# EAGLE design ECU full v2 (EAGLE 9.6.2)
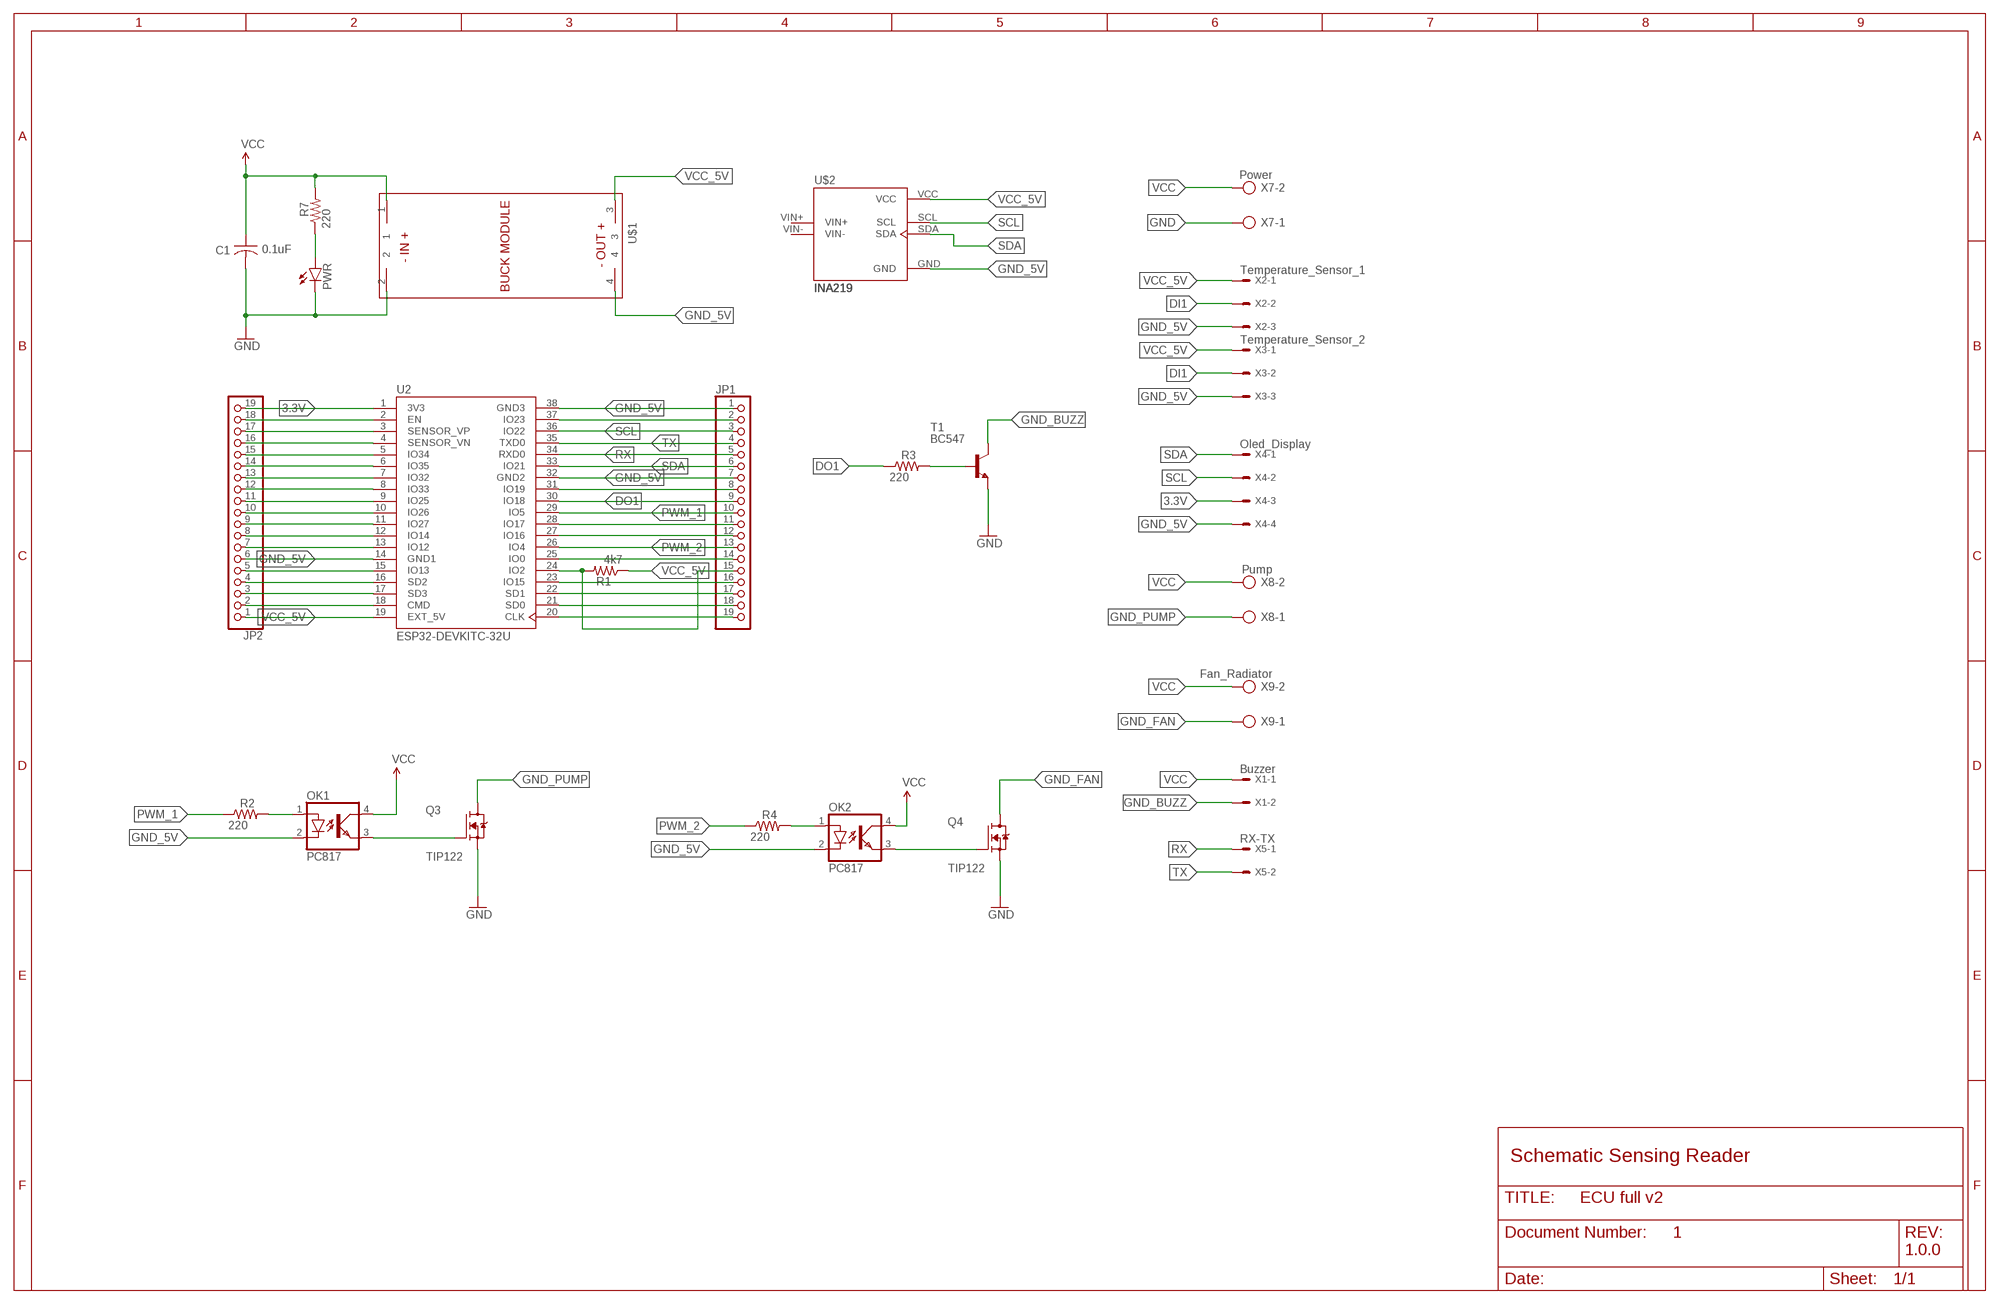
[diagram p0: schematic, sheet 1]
FRAME1 (FRAME_B_L): DESIGNER: PRATIK MAKWANA; DOC: 1; REV: 1.0.0

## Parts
C1  0.1uF  C-US050-030X075  [C050-030X075]
JP1  PINHD-1X19  [1X19]
JP2  PINHD-1X19  [1X19]
OK1  PC817  [DIL04]
OK2  PC817  [DIL04]
PWR  LED5MM  [LED5MM]
Q3  TIP122  IRF3205  [TO254P1041X444X2933-3]
Q4  TIP122  IRF3205  [TO254P1041X444X2933-3]
R1  4k7  R-US_0207/10  [0207/10]
R2  220  R-US_0207/10  [0207/10]
R3  220  R-US_0207/10  [0207/10]
R4  220  R-US_0207/10  [0207/10]
R7  220  R-US_0207/10  [0207/10]
T1  BC547  [TO92]
U2  ESP32-DEVKITC-32U  [MODULE_ESP32-DEVKITC-32U]
U$1  BUCK_MODULEWITH_SMDPADS&THROUGHHOLES  [BUCK_MODULE]
U$2  INA219  [INA219]
X1  Buzzer  22-23-2021  [22-23-2021]
X2  Temperature_Sensor_1  22-23-2031  [22-23-2031]
X3  Temperature_Sensor_2  22-23-2031  [22-23-2031]
X4  Oled_Display  22-23-2041  [22-23-2041]
X5  RX-TX  22-23-2021  [22-23-2021]
X7  Power  AK500/2  [AK500/2]
X8  Pump  AK500/2  [AK500/2]
X9  Fan_Radiator  AK500/2  [AK500/2]

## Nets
3.3V: JP2.19 U2.1(3V3) X4.3
DI1: JP1.15 R1.2 U2.24(IO2) X2.2 X3.2
DO1: JP1.9 R3.1 U2.30(IO18)
GND: C1.2 PWR.K(C) Q3.3(S) Q4.3(S) T1.1(E) U$1.2 X7.1
GND_5V: JP1.1 JP1.7 JP2.6 OK1.2(C) OK2.2(C) U2.14(GND1) U2.32(GND2) U2.38(GND3) U$1.4 U$2.GND X2.3 X3.3 X4.4
GND_BUZZ: T1.3(C) X1.2
GND_FAN: Q4.2(D) X9.1
GND_PUMP: Q3.2(D) X8.1
N$1: OK1.1(A) R2.2
N$2: JP2.18 U2.2(EN)
N$3: JP2.17 U2.3(SENSOR_VP)
N$4: JP2.16 U2.4(SENSOR_VN)
N$5: JP2.15 U2.5(IO34)
N$6: JP2.14 U2.6(IO35)
N$7: JP2.13 U2.7(IO32)
N$8: JP2.12 U2.8(IO33)
N$9: JP2.11 U2.9(IO25)
N$10: JP2.10 U2.10(IO26)
N$11: JP2.9 U2.11(IO27)
N$12: JP2.8 U2.12(IO14)
N$13: JP2.7 U2.13(IO12)
N$14: JP2.5 U2.15(IO13)
N$15: OK1.3(EMIT) Q3.1(G)
N$16: OK2.1(A) R4.2
N$17: OK2.3(EMIT) Q4.1(G)
N$18: JP1.19 U2.20(CLK)
N$19: JP1.18 U2.21(SD0)
N$20: JP1.17 U2.22(SD1)
N$21: JP1.14 U2.25(IO0)
N$22: JP1.16 U2.23(IO15)
N$23: JP1.12 U2.27(IO16)
N$24: JP1.11 U2.28(IO17)
N$25: JP2.2 U2.18(CMD)
N$26: JP1.2 U2.37(IO23)
N$27: JP2.3 U2.17(SD3)
N$28: JP2.4 U2.16(SD2)
N$29: JP1.8 U2.31(IO19)
N$30: PWR.A R7.1
N$33: R3.2 T1.2(B)
PWM_1: JP1.10 R2.1 U2.29(IO5)
PWM_2: JP1.13 R4.1 U2.26(IO4)
RX: JP1.5 U2.34(RXD0) X5.1
SCL: JP1.3 U2.36(IO22) U$2.SCL X4.2
SDA: JP1.6 U2.33(IO21) U$2.SDA X4.1
TX: JP1.4 U2.35(TXD0) X5.2
VCC: C1.1 OK1.4(COL) OK2.4(COL) R7.2 U$1.1 X1.1 X7.2 X8.2 X9.2
VCC_5V: JP2.1 R1.1 U2.19(EXT_5V) U$1.3 U$2.VCC X2.1 X3.1
Unconnected: U$2.VIN+ U$2.VIN-

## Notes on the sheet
- Schematic Sensing Reader

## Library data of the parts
C1 = adafruit:C-US: CAPACITOR, American symbol
JP1 JP2 = pinhead:PINHD-1X19: PIN HEADER
OK1 OK2 = optocoupler:PC817: SHARP OPTO COUPLER; MPN: PC817X4J000F; OC_FARNELL: 9707727; OC_NEWARK: 97K7059
PWR = led:LED: LED
Q3 Q4 = IRF3205:IRF3205: N-Channel 55V 75A (Tc) 170W (Tc) Through Hole TO-220AB Check availability; AVAILABILITY: In Stock; CHECK_PRICES: https://www.snapeda.com/parts/IRF3205/Infineon/view-part/?ref=eda; DESCRIPTION: N-Channel 55V 110A (Tc) 200W (Tc) Through Hole TO-220AB; MF: Infineon Technologies; MP: IRF3205; PACKAGE: TO-220 Infineon; PRICE: None; SNAPEDA_LINK: https://www.snapeda.com/parts/IRF3205/Infineon/view-part/?ref=snap
R1-R4 R7 = adafruit:R-US_: RESISTOR, American symbol
T1 = transistor:BC547: NPN TRANSISTOR
U2 = ESP32-DEVKITC-32U:ESP32-DEVKITC-32U: Check availability; AVAILABILITY: In Stock; CHECK_PRICES: https://www.snapeda.com/parts/ESP32-DEVKITC-32U/Espressif+Systems/view-part/?ref=eda; DESCRIPTION: ESP32-WROOM-32UE series Transceiver; 802.11 b/g/n (Wi-Fi, WiFi, WLAN), Bluetooth® Smart Ready 4.x Dual Mode Evaluation Board; MF: Espressif Systems; MP: ESP32-DEVKITC-32U; PACKAGE: CUSTOM-38 ESPRESSIF; PRICE: None; SNAPEDA_LINK: https://www.snapeda.com/parts/ESP32-DEVKITC-32U/Espressif+Systems/view-part/?ref=snap
U$1 = BUCK_MODULE:BUCK_MODULE
U$2 = INA219:INA219
X1 X5 = con-molex:22-23-2021: .100" (2.54mm) Center Header - 2 Pin; MF: MOLEX; MPN: 22-23-2021; OC_FARNELL: 1462926; OC_NEWARK: 25C3832
X2 X3 = con-molex:22-23-2031: .100" (2.54mm) Center Header - 3 Pin; MF: MOLEX; MPN: 22-23-2031; OC_FARNELL: 1462950; OC_NEWARK: 30C0862
X4 = con-molex:22-23-2041: .100" (2.54mm) Center Header - 4 Pin; MF: MOLEX; MPN: 22-23-2041; OC_FARNELL: 1462920; OC_NEWARK: 38C0355
X7-X9 = con-ptr500:AK500/2: CONNECTOR; OC_FARNELL: unknown; OC_NEWARK: unknown

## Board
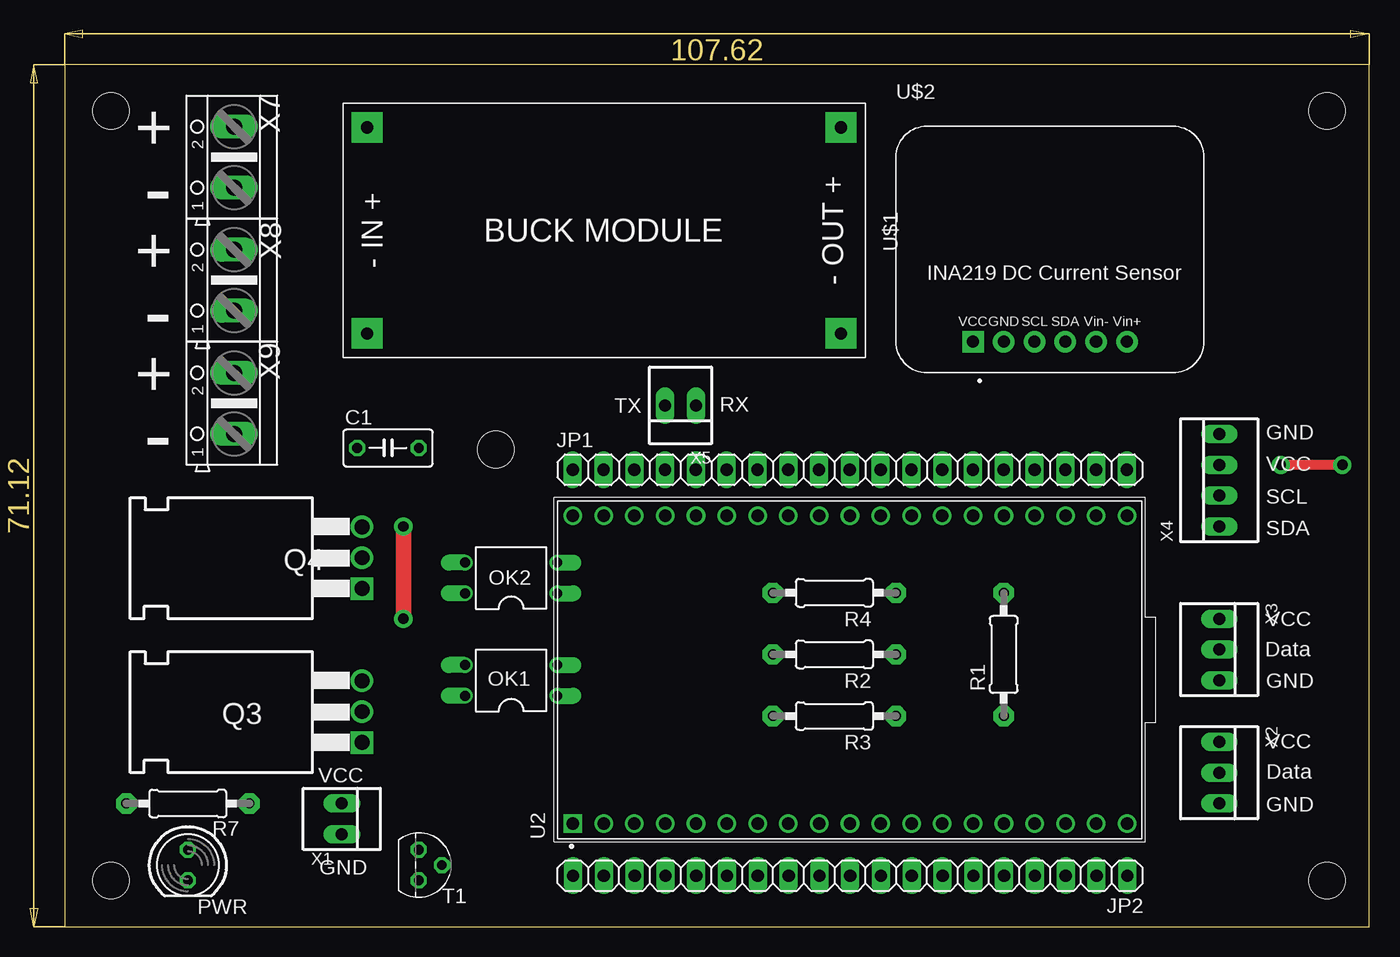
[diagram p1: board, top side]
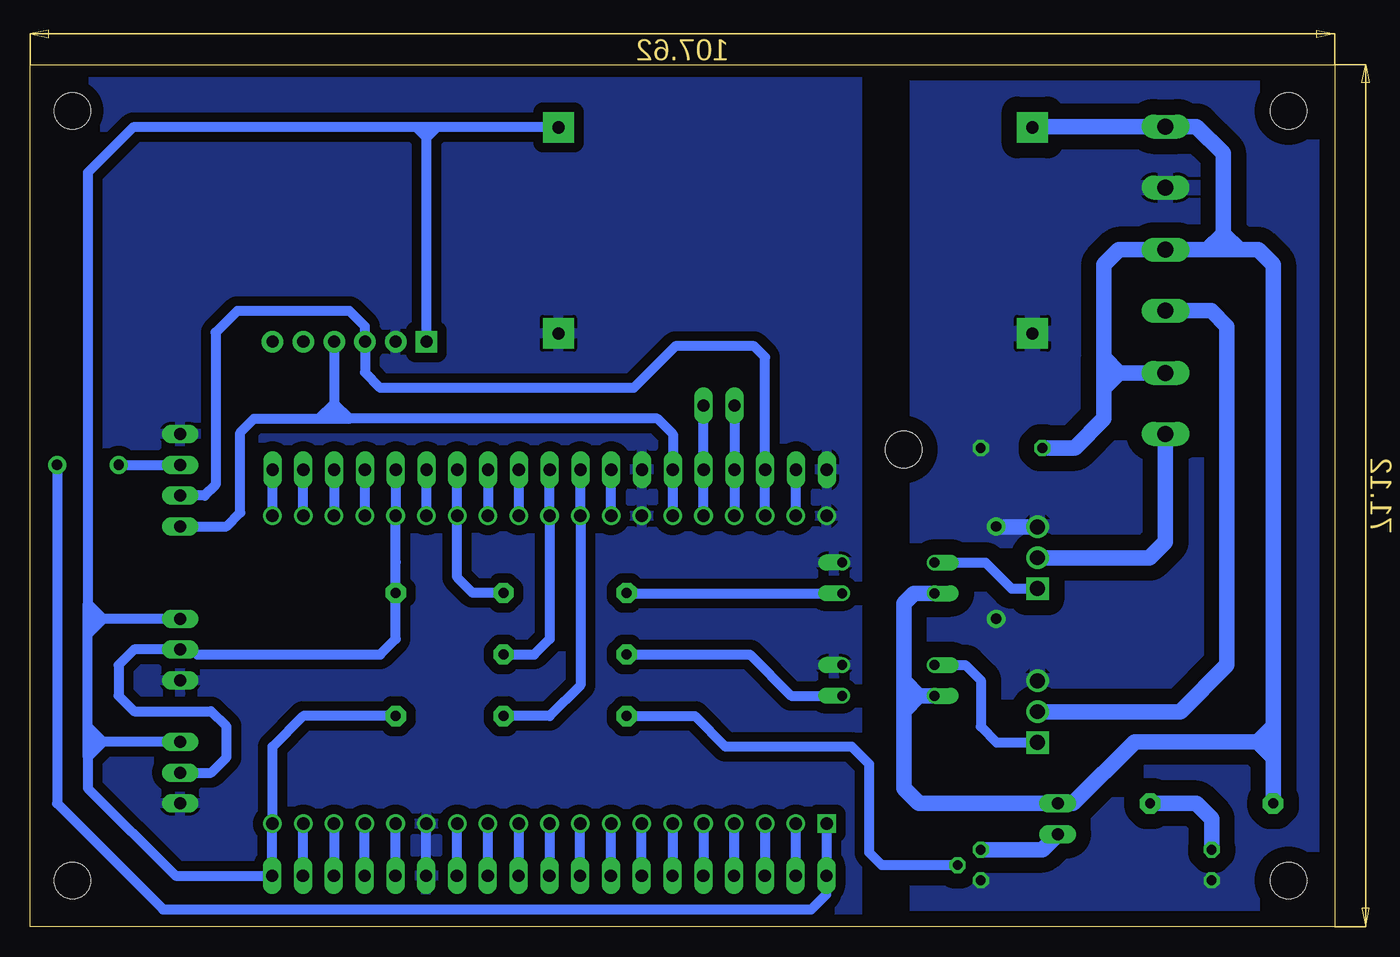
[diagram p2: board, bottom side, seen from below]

Size 110.46 x 73.96 mm. Coordinates in mm from the lower left corner, seen from the top.
Outline: 2.84,0 110.46,0 110.46,71.11 2.84,71.11 2.84,0
Copper layers (1*16): Top 0.035mm / dielectric 1.5mm / Bottom 0.035mm
Design rules "default": minimum track width 6mil, minimum drill 0.35mm, track to track 6mil, track to pad 6mil, pad to pad 6mil, via to via 6mil, smd to smd 6mil, copper to edge 40mil, drill to drill 6mil, minimum pad ring 10mil, minimum via ring 8mil, stop-mask expansion 4mil, vias tented up to drill 0mil, thermal gap 10mil
Holes 3 mm at 106.98,3.81 6.65,67.31 6.65,3.81 106.98,67.31 38.4,39.37

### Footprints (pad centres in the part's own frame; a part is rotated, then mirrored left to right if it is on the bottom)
C050-030X075 = drill 0.813 octagon: 1 -2.54,0; 2 2.54,0
1X19 = drill 1.016 long: 1 -22.86,0; 2 -20.32,0; 3 -17.78,0; 4 -15.24,0; 5 -12.7,0; 6 -10.16,0; 7 -7.62,0; 8 -5.08,0; 9 -2.54,0; 10 0,0; 11 2.54,0; 12 5.08,0; 13 7.62,0; 14 10.16,0; 15 12.7,0; 16 15.24,0; 17 17.78,0; 18 20.32,0; 19 22.86,0
DIL04 = drill 0.813 offset: 1 -1.27,-3.81; 2 1.27,-3.81; 3 1.27,3.81; 4 -1.27,3.81
LED5MM = drill 0.813 octagon: A -1.27,0; K 1.27,0
TO254P1041X444X2933-3 = drill 1.23 pad 1.85 square: 1 2.5,-4.2 | drill 1.23 pad 1.85: 2 5.04,-4.2; 3 7.58,-4.2
0207/10 = drill 0.813 pad 1.676 octagon: 1 -5.08,0; 2 5.08,0
TO92 = drill 0.813 octagon: 1 1.27,0; 2 0,1.905; 3 -1.27,0
MODULE_ESP32-DEVKITC-32U = drill 1.02 square: 1 -12.7,22.85 | drill 1.02: 2 -12.7,20.31; 3 -12.7,17.77; 4 -12.7,15.23; 5 -12.7,12.69; 6 -12.7,10.15; 7 -12.7,7.61; 8 -12.7,5.07; 9 -12.7,2.53; 10 -12.7,-0.01; 11 -12.7,-2.55; 12 -12.7,-5.09; 13 -12.7,-7.63; 14 -12.7,-10.17; 15 -12.7,-12.71; 16 -12.7,-15.25; 17 -12.7,-17.79; 18 -12.7,-20.33; 19 -12.7,-22.87; 20 12.7,-22.87; 21 12.7,-20.33; 22 12.7,-17.79; 23 12.7,-15.25; 24 12.7,-12.71; 25 12.7,-10.17; 26 12.7,-7.63; 27 12.7,-5.09; 28 12.7,-2.55; 29 12.7,-0.01; 30 12.7,2.53; 31 12.7,5.07; 32 12.7,7.61; 33 12.7,10.15; 34 12.7,12.69; 35 12.7,15.23; 36 12.7,17.77; 37 12.7,20.31; 38 12.7,22.85
BUCK_MODULE = drill 1 pad 2.54 square: 1 -8.5,-19.5; 2 8.5,-19.5; 3 -8.5,19.6; 4 8.5,19.6
INA219 = drill 1 pad 1.778: GND 8.89,2.54; SCL 11.43,2.54; SDA 13.97,2.54; VIN+ 19.05,2.54; VIN- 16.51,2.54 | drill 1 pad 1.778 square: VCC 6.35,2.54
22-23-2021 = drill 1 long: 1 -1.27,0; 2 1.27,0
22-23-2031 = drill 1 long: 1 -2.54,0; 2 0,0; 3 2.54,0
22-23-2041 = drill 1 long: 1 -3.81,0; 2 -1.27,0; 3 1.27,0; 4 3.81,0
AK500/2 = drill 1.321 long: 1 -2.515,0; 2 2.515,0

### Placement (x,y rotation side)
C1  29.51,39.5 0 top
JP1  67.61,37.7 0 top
JP2  67.64,4.2 180 top
OK1  39.67,20.32 90 top
OK2  39.67,28.77 90 top
PWR  13,5.08 270 top
Q3  23.16,12.7 90 top
Q4  23.16,25.4 90 top
R1  80.31,22.46 90 top
R2  66.34,22.46 180 top
R3  66.34,17.38 180 top
R4  66.34,27.54 180 top
R7  13,10.16 180 top
T1  32.05,5.08 270 top
U2  67.61,21.19 90 top
U$1  47.29,57.45 270 top
U$2  71.42,45.72 0 top
X1  25.7,8.89 270 top
X2  98.09,12.7 270 top
X3  98.09,22.86 270 top
X4  98.09,36.83 90 top
X5  53.64,43 180 top
X7  16.81,63.5 90 top
X8  16.81,53.34 90 top
X9  16.81,43.18 90 top

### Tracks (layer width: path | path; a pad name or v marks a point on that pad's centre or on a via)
3.3V  (via drill 0.85 pad 1.5)
  Top 0.813: v108.25,38.1 v103.17,38.1
  Bottom 0.813: v103.17,38.1 X4.3 | v108.25,38.1 108.25,10.16 99.51,1.42 46.02,1.42 44.78,2.66 JP2.19 44.78,8.47 U2.1
DI1
  Bottom 0.813: JP1.15 U2.24 R1.2 | R1.2 80.31,30.08 | X2.2 95.55,12.7 94.28,13.97 94.28,16.51 95.55,17.78 101.9,17.78 103.17,19.05 103.17,21.59 101.9,22.86 X3.2 97.09,22.86 96.69,22.46 81.58,22.46 80.31,23.73 R1.2
DO1
  Bottom 0.813: JP1.9 U2.30 65.08,19.91 67.61,17.38 R3.1
GND  (via drill 0.85 pad 1.5)
  Top 1.27: v30.78,33.02 v30.78,25.4
  Bottom 1.27: Q4.3 30.74,32.98 v30.78,33.02
  pour Bottom (isolate 1.27): 2.84,71.12 37.26,71.12 37.26,0 2.84,0
GND_5V
  Bottom 0.813: JP2.6 77.8,8.47 U2.14
  pour Bottom (isolate 0.813): 110.79,71.12 110.79,0 42.21,0 42.21,71.12
GND_BUZZ
  Bottom 1.27: T1.3 26.97,6.35 X1.2
GND_FAN
  Bottom 1.27: X9.1 16.81,31.75 18.12,30.44 Q4.2
GND_PUMP
  Bottom 1.27: X8.1 13.03,50.83 11.73,49.53 11.73,21.59 15.58,17.74 Q3.2
N$1
  Bottom 0.813: R2.2 51.1,22.46 47.69,19.05 OK1.1
N$2
  Bottom 0.813: JP2.18 47.3,4.22 U2.2
N$3
  Bottom 0.813: U2.3 49.84,4.22 JP2.17
N$4
  Bottom 0.813: JP2.16 52.38,4.22 U2.4
N$5
  Bottom 0.813: U2.5 54.94,8.47 JP2.15
N$6
  Bottom 0.813: U2.6 57.48,8.47 JP2.14
N$7
  Bottom 0.813: JP2.13 60.02,8.47 U2.7
N$8
  Bottom 0.813: JP2.12 62.56,8.47 U2.8
N$9
  Bottom 0.813: JP2.11 65.1,8.47 U2.9
N$10
  Bottom 0.813: U2.10 67.62,4.22 JP2.10
N$11
  Bottom 0.813: U2.11 70.18,8.47 JP2.9
N$12
  Bottom 0.813: U2.12 72.72,8.47 JP2.8
N$13
  Bottom 0.813: JP2.7 75.26,8.47 U2.13
N$14
  Bottom 0.813: U2.15 80.34,8.47 JP2.5
N$15
  Bottom 0.813: OK1.3 33.32,21.59 32.05,20.32 32.05,16.51 30.74,15.2 Q3.1
N$16
  Bottom 0.813: R4.2 61.22,27.5 OK2.1
N$17
  Bottom 0.813: OK2.3 31.65,30.04 29.51,27.9 Q4.1
N$18
  Bottom 0.813: U2.20 JP1.19
N$19
  Bottom 0.813: U2.21 JP1.18
N$20
  Bottom 0.813: JP1.17 U2.22
N$21
  Bottom 0.813: U2.25 JP1.14
N$22
  Bottom 0.813: U2.23 JP1.16
N$23
  Bottom 0.813: JP1.12 U2.27
N$24
  Bottom 0.813: U2.28 JP1.11
N$25
  Bottom 0.813: JP2.2 87.96,8.47 U2.18
N$26
  Bottom 0.813: U2.37 JP1.2
N$27
  Bottom 0.813: U2.17 85.4,4.22 JP2.3
N$28
  Bottom 0.813: JP2.4 82.88,8.47 U2.16
N$29
  Bottom 0.813: U2.31 JP1.8
N$30
  Bottom 1.27: PWR.A 13,8.89 14.27,10.16 R7.1
N$33
  Bottom 0.813: R3.2 55.63,17.38 53.09,14.84 42.68,14.84 41.24,13.4 41.24,6.1 40.22,5.08 T1.2
PWM_1
  Bottom 0.813: JP1.10 U2.29 67.62,23.72 68.88,22.46 R2.1
PWM_2
  Bottom 0.813: JP1.13 U2.26 75.24,28.82 73.96,27.54 R4.1
RX
  Bottom 0.813: U2.34 JP1.5 X5.1
SCL
  Bottom 0.813: U2.36 JP1.3 49.83,46.99 50.74,47.9 57.24,47.9 60.69,44.45 81.58,44.45 82.85,45.72 U$2.SCL 82.85,49.53 84.12,50.8 93.39,50.8 95.17,49.02 95.17,36.45 96.06,35.56 X4.2
SDA
  Bottom 0.813: U2.33 JP1.6 57.45,40.64 58.72,41.91 84.12,41.91 | 84.12,41.91 85.39,43.18 | U$2.SDA 85.39,43.18 | X4.1 94.28,33.02 93.14,34.16 93.14,40.77 91.99,41.91 86.66,41.91 | 86.66,41.91 85.39,41.91 | 85.39,41.91 84.12,41.91 | 85.39,43.18 86.66,41.91 | 85.39,43.18 85.39,41.91
TX
  Bottom 0.813: U2.35 JP1.4 X5.2
VCC
  Bottom 1.27: OK2.4 37.57,27.5 38.4,26.67 38.4,20.32 | 21.89,46.99 21.89,54.61 20.64,55.85 X8.2 13.38,55.85 | 21.89,46.99 20.59,45.7 | X9.2 20.59,45.7 | 16.79,66.04 X7.2 | X7.2 14.24,66.02 12.04,63.81 12.04,57.2 | OK1.4 37.13,19.05 | 38.4,20.32 37.13,19.05 | 7.92,16.51 7.92,54.61 9.16,55.85 10.7,55.85 | 7.92,16.51 7.92,13.97 | 7.92,13.97 R7.2 | 9.19,15.24 7.92,16.51 | 9.19,15.24 7.92,13.97 | 9.19,15.24 19.35,15.24 24.43,10.16 X1.1 37.13,10.16 38.4,11.43 38.4,17.78 | C1.1 24.3,39.5 21.89,41.91 21.89,44.45 | 21.89,44.45 21.89,46.99 | 20.59,45.7 20.64,45.7 21.89,44.45 | 38.4,17.78 38.4,20.32 | 37.13,19.05 38.4,17.78 | X7.2 27.73,66.02 U$1.1 | 13.38,55.85 12.04,55.85 | 12.04,55.85 10.7,55.85 | 12.04,55.85 12.04,57.2 | 12.04,57.2 10.7,55.85 | 12.04,57.2 13.38,55.85
VCC_5V
  Bottom 0.813: R1.1 87.94,17.38 90.48,14.84 U2.19 90.5,8.47 JP2.1 98.48,4.2 105.71,11.43 105.71,13.97 | 105.71,16.51 105.71,24.13 | X2.1 104.44,15.24 | 105.71,16.51 104.44,15.24 | X3.1 104.44,25.4 | 105.71,24.13 104.44,25.4 | 105.71,24.13 105.71,25.4 | 105.71,25.4 105.71,26.67 | 104.44,25.4 105.71,26.67 | 104.44,25.4 105.71,25.4 | 105.71,26.67 105.71,62.23 101.99,65.95 78.64,65.95 | 105.71,13.97 105.71,15.24 | 105.71,15.24 105.71,16.51 | 104.44,15.24 105.71,13.97 | 104.44,15.24 105.71,15.24 | U$1.3 76.9,65.95 | 76.9,65.95 78.64,65.95 | 78.64,65.95 77.77,65.08 | U$2.VCC 77.77,65.08 | 77.77,65.08 76.9,65.95

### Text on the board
tPlace: + | - | + | - | + | TX | RX | - | GND | VCC | SCL | SDA | VCC | Data | GND | VCC | Data | VCC | GND | GND

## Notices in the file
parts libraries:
SparkFun: Licensing: CC v3.0 Share-Alike You are welcome to use this library for commercial purposes.
